FUNCTION_BLOCK p07_ST_motor
VAR_INPUT
	forward: BOOL;
	backward: BOOL;
	lockTime: TIME;
END_VAR
VAR_OUTPUT
	movement: BOOL;
	direction: BOOL;
END_VAR
VAR
	forwardTimer: TOF;
	backwardTimer: TOF;
	rotateForward: BOOL;
	rotateBackward: BOOL;
	backwardLock: BOOL;
	forwardLock: BOOL;
END_VAR

// Call of the timer function blocks
forwardTimer(IN:=forward, PT:=lockTime, Q => backwardLock);
backwardTimer(IN:=backward, PT:=lockTime, Q => forwardLock);

// Calculation of whether the motor can rotate forward or backward
rotateForward := forward AND NOT forwardLock;
rotateBackward := backward AND NOT backwardLock;

// Output movement
movement := rotateForward OR rotateBackward;

// Output direction - we want to save the relay for direction,
// so we will store the state of the direction.
(* 
IF rotateBackward THEN
	direction := TRUE;
ELSIF rotateForward THEN
	direction := FALSE;
ELSE               			  // This can
	direction := direction;  // be omitted.
END_IF
*)

// Shorter:
IF movement THEN
	direction := rotateBackward;
END_IF

END_FUNCTION_BLOCK
